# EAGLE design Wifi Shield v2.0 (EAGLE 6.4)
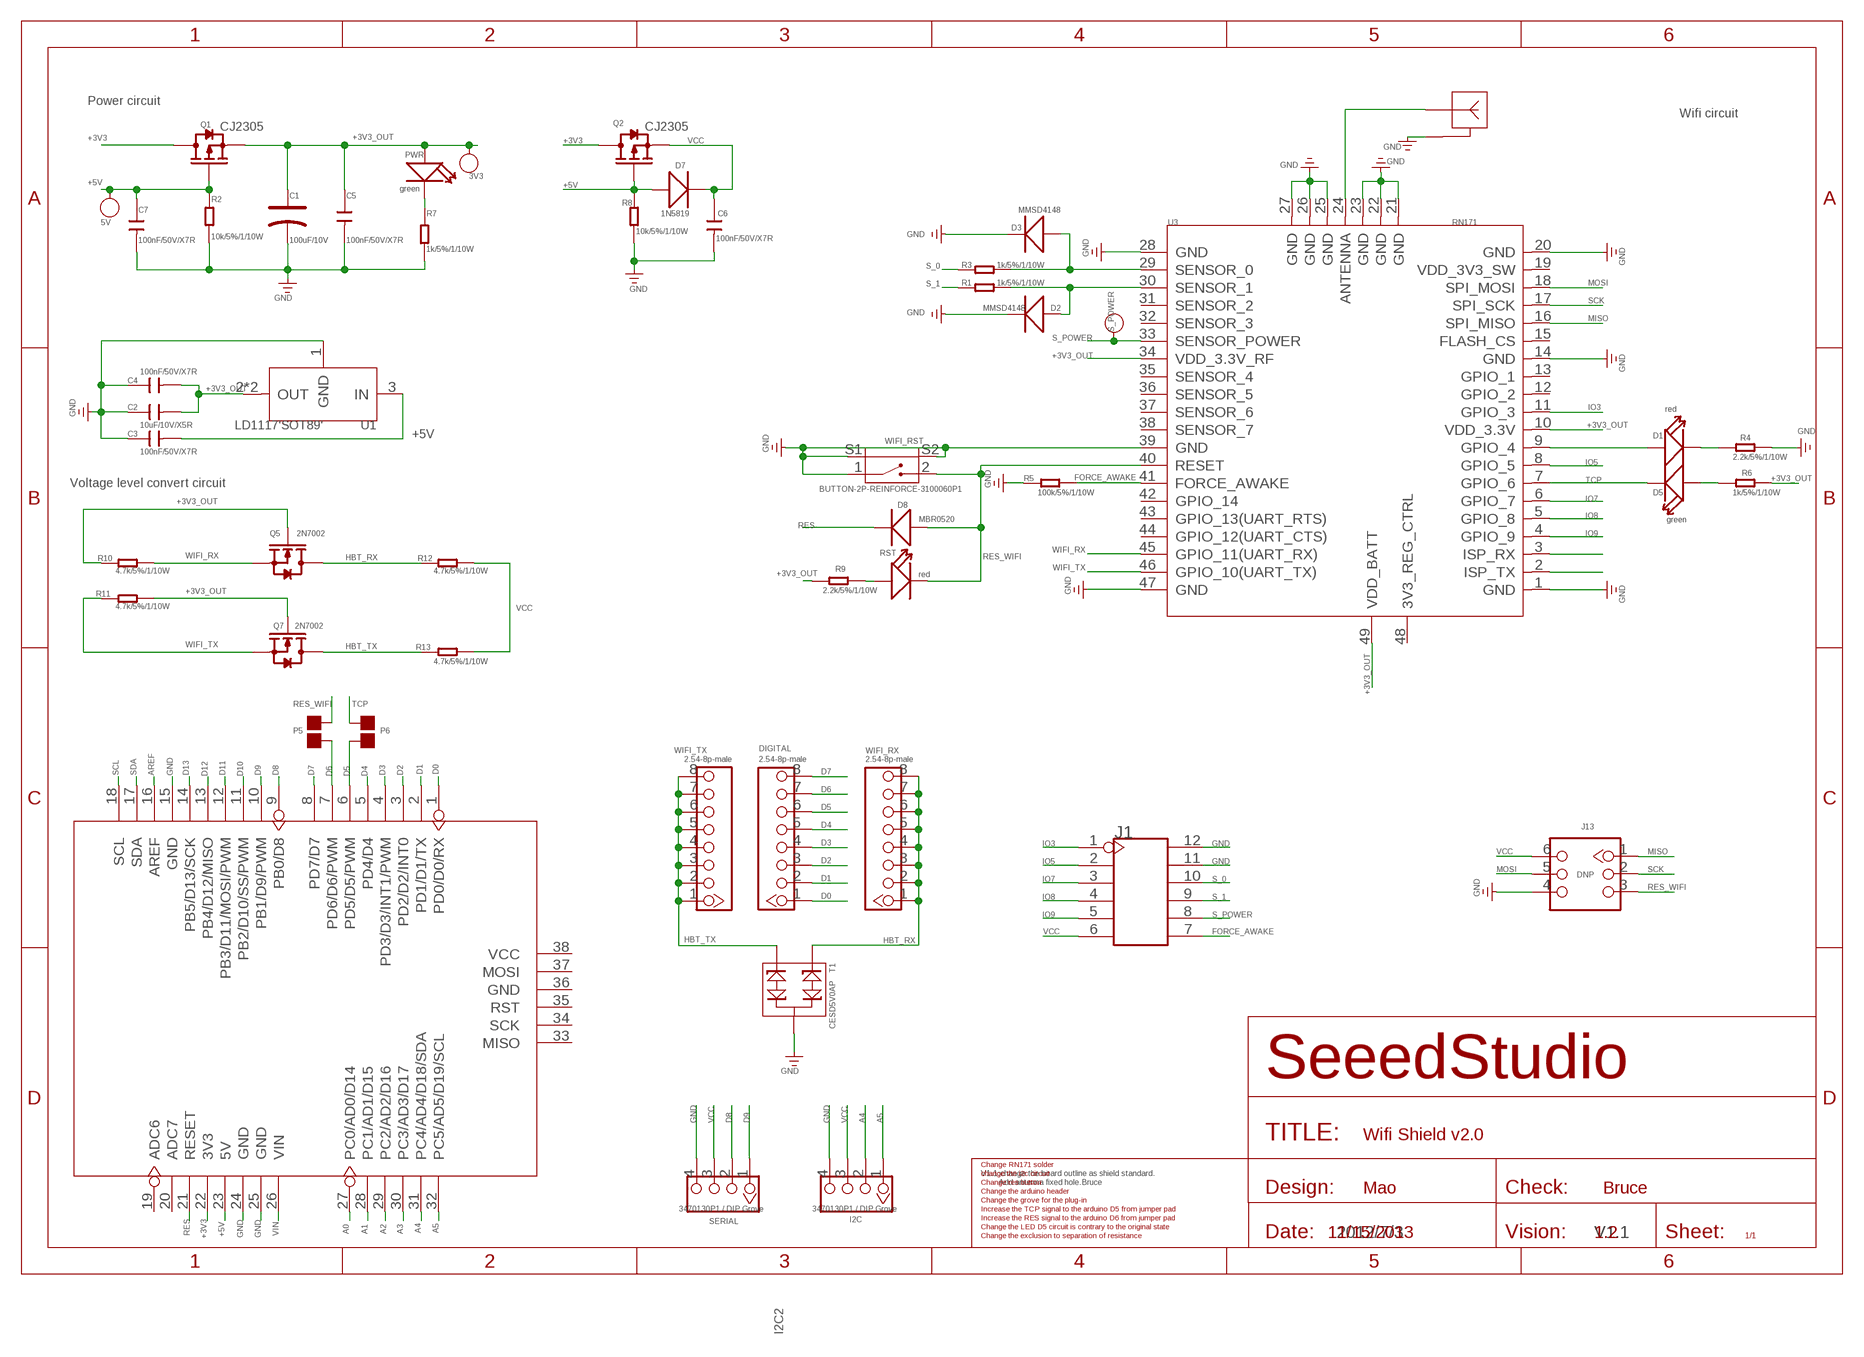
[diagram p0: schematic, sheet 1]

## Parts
3V3  PAD-TEST-POINT'4545'  [TP_4545]
5V  PAD-TEST-POINT'4545'  [TP_4545]
ANT3  2.4G-ANTNORMAL  [2.4G-ANT]
C1  100uF/10V  CAP-AVX-B  [AVX-B]
C2  10uF/10V/X5R  C-0805  [C0805]
C3  100nF/50V/X7R  C-0603  [C0603]
C4  100nF/50V/X7R  C-0603  [C0603]
C5  100nF/50V/X7R  C-0603  [C0603]
C6  100nF/50V/X7R  C-0603  [C0603]
C7  100nF/50V/X7R  C-0603  [C0603]
D1  red  LED'0603'  [LED-0603]
D2  MMSD4148  D'MBR0520LT1'  [SOD123-2.7X1.6]
D3  MMSD4148  D'MBR0520LT1'  [SOD123-2.7X1.6]
D5  green  LED'0603'  [LED-0603]
D7  1N5819  D'DO-214AC'  [D2010]
D8  MBR0520  D'MBR0520LT1'  [SOD123-2.7X1.6]
DIGITAL  2.54-8p-male  HEADER-8P-2.54  [8P-2.54]
I2C  3470130P1 / DIP Grove  TWIG-4P-2.0-2.0  [4P-2.0]
J1  HEADER-2X6P-2.54  [2X6P-2.54]
J13  DNP  HEADER-2X3P-2.54  [2X3P-2.54]
P5  DNP  PAD-JUMPER-2P  [2P-SMD-1.78X1.27]
P6  DNP  PAD-JUMPER-2P  [2P-SMD-1.78X1.27]
PWR  green  LED'0603'  [LED-0603]
Q1  CJ2305  MOSFET-P'SI2323CDS/SI2305DS<BR>'  [SOT23]
Q2  CJ2305  MOSFET-P'SI2323CDS/SI2305DS<BR>'  [SOT23]
Q5  2N7002  MOSFET-N'SOT23'  [SOT23]
Q7  2N7002  MOSFET-N'SOT23'  [SOT23]
R1  1k/5%/1/10W  R-0603  [R0603]
R2  10k/5%/1/10W  R-0603  [R0603]
R3  1k/5%/1/10W  R-0603  [R0603]
R4  2.2k/5%/1/10W  R-0603  [R0603]
R5  100k/5%/1/10W  R-0603  [R0603]
R6  1k/5%/1/10W  R-0603  [R0603]
R7  1k/5%/1/10W  R-0603  [R0603]
R8  10k/5%/1/10W  R-0603  [R0603]
R9  2.2k/5%/1/10W  R-0603  [R0603]
R10  4.7k/5%/1/10W  R-0603  [R0603]
R11  4.7k/5%/1/10W  R-0603  [R0603]
R12  4.7k/5%/1/10W  R-0603  [R0603]
R13  4.7k/5%/1/10W  R-0603  [R0603]
RST  red  LED'0603'  [LED-0603]
S_POWER  PAD-TEST-POINT'4545'  [TP_4545]
SERIAL  3470130P1 / DIP Grove  TWIG-4P-2.0-2.0  [4P-2.0]
T1  CESD5V0AP  D-ESD-PESDXL2BT  [SOT23]
U1  LD1117'SOT89'  [SOT89]
U3  RN171  WIFI-RN-171  [49P-1.27-26.67X17.78]
U6  ARDUINO-38P  [ARDUINO-38P-WITH/-SILK]
WIFI_RST  BUTTON-2P-REINFORCE-3100060P1  [4P-SMD-7.0X3.5X3.5H-90D]
WIFI_RX  2.54-8p-male  HEADER-8P-2.54  [8P-2.54]
WIFI_TX  2.54-8p-male  HEADER-8P-2.54  [8P-2.54]

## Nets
+3V3: Q1.3(D) Q2.3(D) U6.22(3V3)
+3V3_OUT: 3V3.T C1.+ C2.2 C4.2 C5.1 PWR.+ Q1.2(S) Q5.1(G) Q7.1(G) R6.1 R9.2 R10.2 R11.1 U1.2(OUT) U1.4(OUT) U3.10(VDD_3.3V) U3.34(VDD_3.3V_RF) U3.49(VDD_BATT)
+5V: 5V.T C3.2 C7.1 D7.+ Q1.1(G) Q2.1(G) R2.1 R8.1 U1.3(IN) U6.23(5V)
A0: U6.27(PC0/AD0/D14)
A1: U6.28(PC1/AD1/D15)
A2: U6.29(PC2/AD2/D16)
A3: U6.30(PC3/AD3/D17)
A4: I2C.2 U6.31(PC4/AD4/D18/SDA)
A5: I2C.1 U6.32(PC5/AD5/D19/SCL)
AREF: U6.16(AREF)
D0: DIGITAL.1 U6.1(PD0/D0/RX)
D1: DIGITAL.2 U6.2(PD1/D1/TX)
D2: DIGITAL.3 U6.3(PD2/D2/INT0)
D3: DIGITAL.4 U6.4(PD3/D3/INT1/PWM)
D4: DIGITAL.5 U6.5(PD4/D4)
D5: DIGITAL.6 P6.2 U6.6(PD5/D5/PWM)
D6: DIGITAL.7 P5.1 U6.7(PD6/D6/PWM)
D7: DIGITAL.8 U6.8(PD7/D7)
D8: SERIAL.2 U6.9(PB0/D8)
D9: SERIAL.1 U6.10(PB1/D9/PWM)
D10: U6.11(PB2/D10/SS/PWM)
D11: U6.12(PB3/D11/MOSI/PWM)
D12: U6.13(PB4/D12/MISO)
D13: U6.14(PB5/D13/SCK)
FORCE_AWAKE: J1.7 R5.1 U3.41(FORCE_AWAKE)
GND: ANT3.1 C1.- C2.1 C3.1 C4.1 C5.2 C6.2 C7.2 D2.2(-) D3.2(-) I2C.4 J1.11 J1.12 J13.4 R2.2 R4.1 R5.2 R7.1 R8.2 SERIAL.4 T1.3 U1.1(GND) U3.1(GND) U3.14(GND) U3.20(GND) U3.21(GND) U3.22(GND) U3.23(GND) U3.25(GND) U3.26(GND) U3.27(GND) U3.28(GND) U3.39(GND) U3.47(GND) U6.15(GND) U6.24(GND) U6.25(GND) WIFI_RST.1 WIFI_RST.S1 WIFI_RST.S2
HBT_RX: Q5.3(D) R12.2 T1.1 WIFI_RX.1 WIFI_RX.2 WIFI_RX.3 WIFI_RX.4 WIFI_RX.5 WIFI_RX.6 WIFI_RX.7 WIFI_RX.8
HBT_TX: Q7.3(D) R13.2 T1.2 WIFI_TX.1 WIFI_TX.2 WIFI_TX.3 WIFI_TX.4 WIFI_TX.5 WIFI_TX.6 WIFI_TX.7 WIFI_TX.8
IO3: J1.1 U3.11(GPIO_3)
IO5: J1.2 U3.8(GPIO_5)
IO7: J1.3 U3.6(GPIO_7)
IO8: J1.4 U3.5(GPIO_8)
IO9: J1.5 U3.4(GPIO_9)
MISO: J13.1 U3.16(SPI_MISO)
MOSI: J13.5 U3.18(SPI_MOSI)
N$1: R9.1 RST.+
N$2: D3.1(+) R3.1 U3.29(SENSOR_0)
N$3: D2.1(+) R1.1 U3.30(SENSOR_1)
N$4: D5.+ R6.2
N$6: ANT3.2 U3.24(ANTENNA)
N$10: U3.2(ISP_TX)
N$11: U3.3(ISP_RX)
N$22: D1.+ U3.9(GPIO_4)
N$25: D1.- R4.2
N$26: PWR.- R7.2
RES: D8.2(-) U6.21(RESET)
RES_WIFI: D8.1(+) J13.3 P5.2 RST.- U3.40(RESET) WIFI_RST.2
S_0: J1.10 R3.2
S_1: J1.9 R1.2
S_POWER: J1.8 S_POWER.T U3.33(SENSOR_POWER)
SCK: J13.2 U3.17(SPI_SCK)
SCL: U6.18(SCL)
SDA: U6.17(SDA)
TCP: D5.- P6.1 U3.7(GPIO_6)
VCC: C6.1 D7.- I2C.3 J1.6 J13.6 Q2.2(S) R12.1 R13.1 SERIAL.3
VIN: U6.26(VIN)
WIFI_RX: Q5.2(S) R10.1 U3.45(GPIO_11(UART_RX))
WIFI_TX: Q7.2(S) R11.2 U3.46(GPIO_10(UART_TX))
Unconnected: U3.12(GPIO_2) U3.13(GPIO_1) U3.15(FLASH_CS) U3.19(VDD_3V3_SW) U3.31(SENSOR_2) U3.32(SENSOR_3) U3.35(SENSOR_4) U3.36(SENSOR_5) U3.37(SENSOR_6) U3.38(SENSOR_7) U3.42(GPIO_14) U3.43(GPIO_13(UART_RTS)) U3.44(GPIO_12(UART_CTS)) U3.48(3V3_REG_CTRL) U6.19(ADC6) U6.20(ADC7) U6.33(MISO) U6.34(SCK) U6.35(RST) U6.36(GND) U6.37(MOSI) U6.38(VCC)

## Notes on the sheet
- Power circuit
- Wifi circuit
- Voltage level convert circuit
- Change RN171 solder
- change the i2c circuit | V1.1:change the board outline as shield standard.
- Change res button | Add antenna fixed hole.Bruce
- Change the arduino header | Mao | Bruce
- Change the grove for the plug-in
- Increase the TCP signal to the arduino D5 from jumper pad
- Increase the RES signal to the arduino D6 from jumper pad
- Change the LED D5 circuit is contrary to the original state
- Change the exclusion to separation of resistance | 11/15/2013 | 2012/7/3 | 1.2 | V1.1
- I2C2

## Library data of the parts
3V3 5V S_POWER = Discrete:PAD-TEST-POINT; PARTNO: DNP
ANT3 = template:2.4G-ANT
C1 = Discrete:CAP*: Electrolytic Capacitors,Tantalum Capacitors and Super Capacitors
C2-C7 = Discrete:C*: Ceramic Capacitors
D1 D5 PWR RST = Discrete:LED*
D2 D3 D7 D8 = Discrete:D*
DIGITAL WIFI_RX WIFI_TX = Connector:HEADER-8P
I2C SERIAL = Connector:TWIG-4P-2.0
J1 = Connector :HEADER-2X6P
J13 = Connector:HEADER-2X3P
P5 P6 = Discrete:PAD-JUMPER-2P; PARTNO: DNP
Q1 Q2 = Discrete:MOSFET-P
Q5 Q7 = Discrete:MOSFET-N: IRLL014: http://www.vishay.com/docs/91319/sihll014.pdf
R1-R13 = Discrete:R*
T1 = Discrete:D-ESD-PESDXL2BT
U1 = IC:LD1117: Low Drop Fixed And Adjustable Positive Voltage Regulators http://www.datasheetcatalog.org/datasheet/SGSThomsonMicroelectronics/mXuqtqv.pdf
U3 = moudle:WIFI-RN-171: WIFLY GSX 802.11 b/g wireless LAN Module
U6 = moudle:ARDUINO-38P
WIFI_RST = Discrete:BUTTON-2P-REINFORCE: TS-1188E http://www.best-dz.com/?thread-374-2.html SMD Button

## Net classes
0 default: width 0.003 mm, drill 0.254 mm, clearance 0.152 mm

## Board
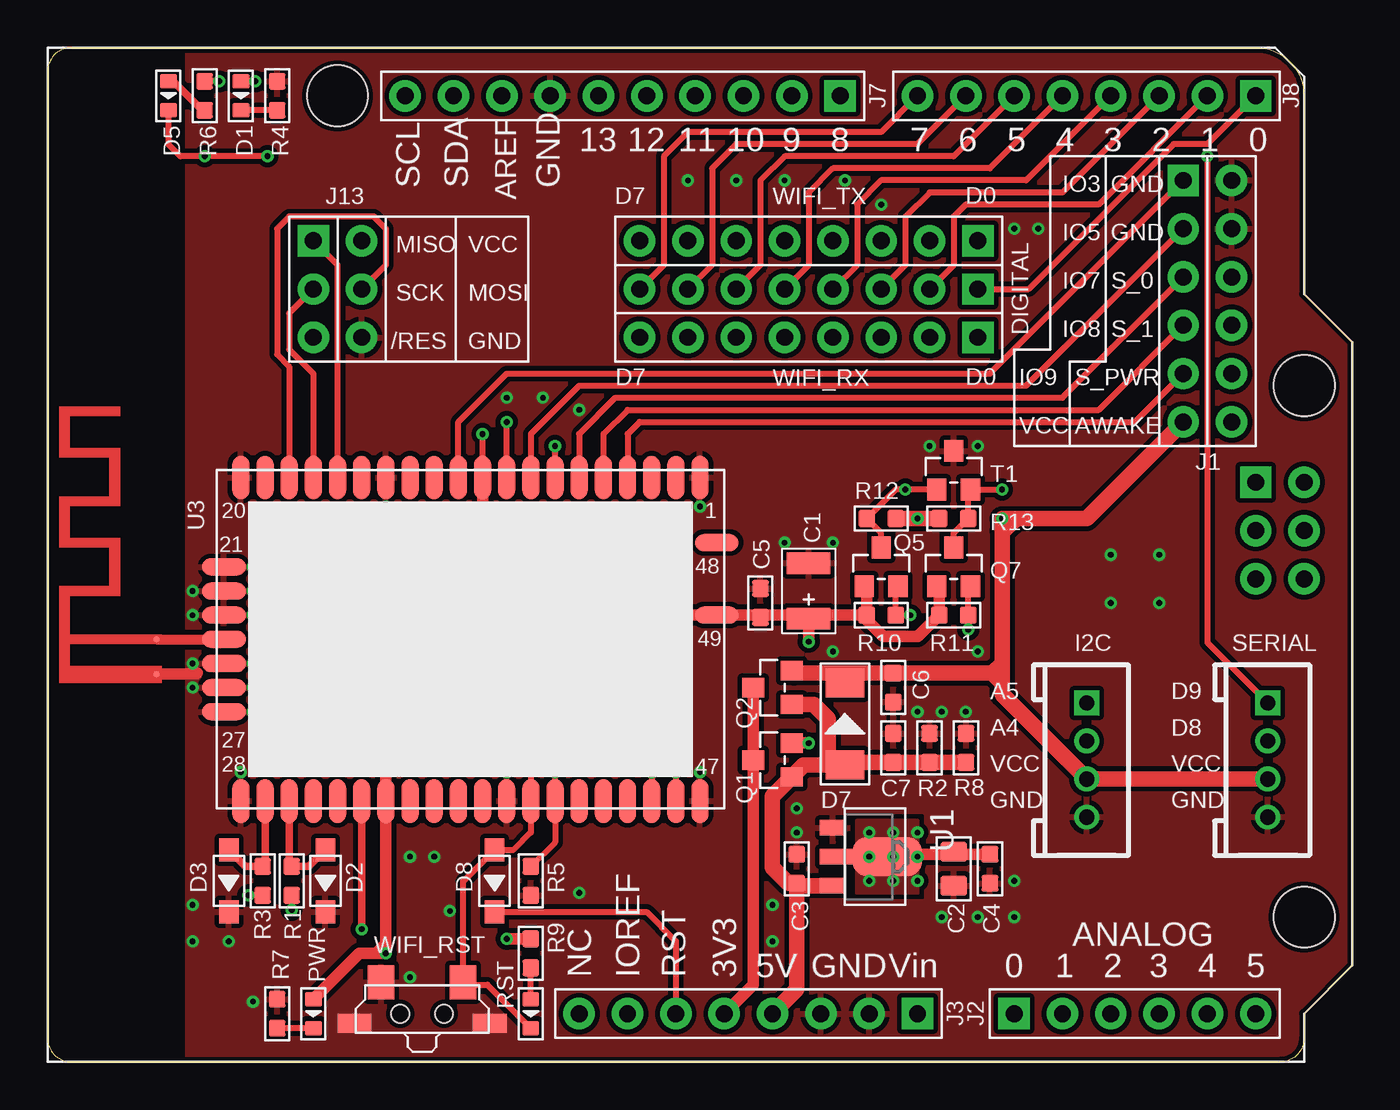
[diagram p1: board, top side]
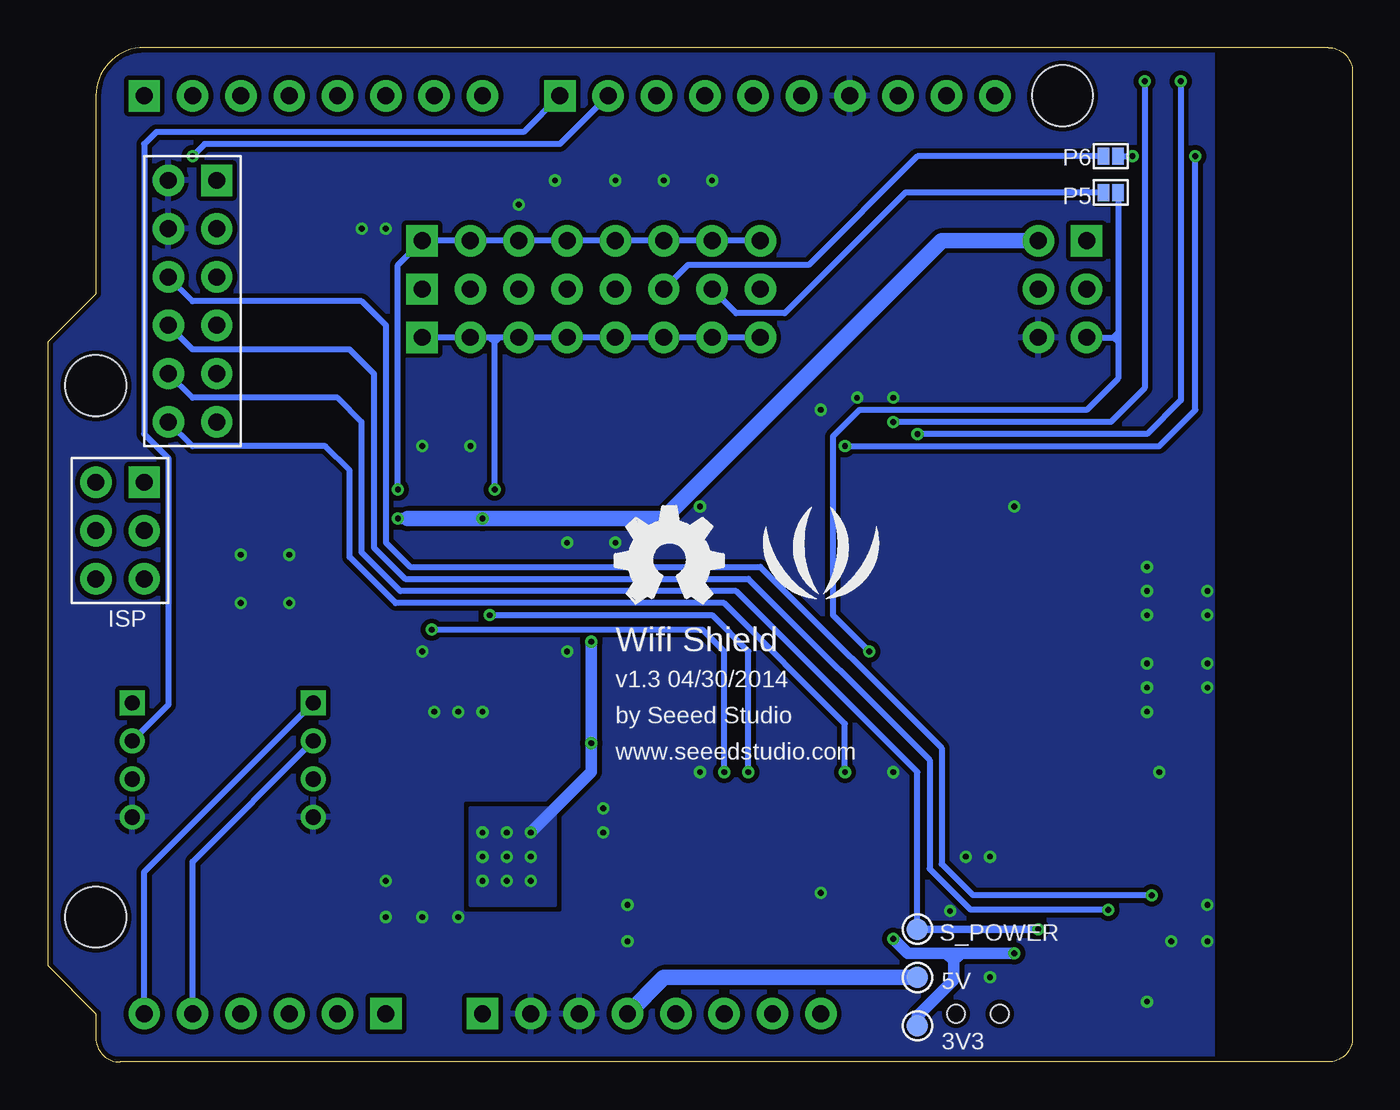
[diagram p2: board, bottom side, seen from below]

Size 68.58 x 53.34 mm. Coordinates in mm from the lower left corner, seen from the top.
Outline: 1.27,53.34 63.5,53.34 arc-90 66.04,50.8 66.04,40.39 68.58,37.85 68.58,5.08 66.04,2.54 66.04,1.27 arc-90 64.77,0 1.27,0 arc-90 0,1.27 0,52.07 arc-90 1.27,53.34
Copper layers (1*16): Top 0.035mm / dielectric 1.5mm / Bottom 0.035mm
Design rules "default": minimum track width 6mil, minimum drill 12mil, track to track 6mil, track to pad 6mil, pad to pad 6mil, via to via 6mil, smd to smd 0mil, copper to edge 10mil, drill to drill 10mil, minimum pad ring 10mil, minimum via ring 6mil, stop-mask expansion 2mil, vias tented up to drill 32mil, thermal gap 10mil
tRestrict: area 0,0 to 7,53.3; area 8.6,17.9 to 9.9,21.7
bRestrict: area 0,0 to 7,53.3

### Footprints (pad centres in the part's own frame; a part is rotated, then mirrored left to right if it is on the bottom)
TP_4545 = smd 1.143 x 1.143: T 0,0
2.4G-ANT = smd 0.305 x 0.305: 1 0.457,0.254; 2 2.286,0.254
AVX-B = smd 1.143 x 2.286: + -1.46,0; - 1.46,0
C0805 = smd 1.016 x 1.397: 1 -0.889,0; 2 0.889,0
C0603 = smd 0.889 x 0.889: 1 -0.762,0; 2 0.762,0
LED-0603 = smd 0.762 x 0.889: + -0.762,0; - 0.762,0
SOD123-2.7X1.6 = smd 1.2 x 1.02: 1 -1.635,0; 2 1.635,0
D2010 = smd 1.524 x 2.032: + -2.159,0; - 2.159,0
8P-2.54 = drill 0.889 pad 1.651 square: 1 0,8.89 | drill 0.889 pad 1.651: 2 0,6.35; 3 0,3.81; 4 0,1.27; 5 0,-1.27; 6 0,-3.81; 7 0,-6.35; 8 0,-8.89
4P-2.0 = drill 0.8 pad 1.27 square: 1 -3,0 | drill 0.8 pad 1.27: 2 -1,0; 3 1,0; 4 3,0
2X6P-2.54 = drill 0.889 pad 1.651 square: 1 -1.27,6.35 | drill 0.889 pad 1.651: 2 -1.27,3.81; 3 -1.27,1.27; 4 -1.27,-1.27; 5 -1.27,-3.81; 6 -1.27,-6.35; 7 1.27,-6.35; 8 1.27,-3.81; 9 1.27,-1.27; 10 1.27,1.27; 11 1.27,3.81; 12 1.27,6.35
2X3P-2.54 = drill 0.889 pad 1.651 square: 1 -1.27,2.54 | drill 0.889 pad 1.651: 2 -1.27,0; 3 -1.27,-2.54; 4 1.27,-2.54; 5 1.27,0; 6 1.27,2.54
2P-SMD-1.78X1.27 = smd 0.889 x 0.61: 1 0,0.381; 2 0,-0.381
SOT23 = smd 1.016 x 1.143: 1 -0.889,-1.016; 2 0.889,-1.016; 3 0,1.016
R0603 = smd 0.889 x 0.889: 1 -0.762,0; 2 0.762,0
SOT89 = smd 0.8 x 1.4: 1 -1.524,-1.905; 3 1.524,-1.905 | smd 0.8 x 1.9: 2 0,-1.651 | smd 2.032 x 3.65: 4 0,0.94
49P-1.27-26.67X17.78 = smd 0.889 x 2.286: 1 12.065,8.509; 2 10.795,8.509; 3 9.525,8.509; 4 8.255,8.509; 5 6.985,8.509; 6 5.715,8.509; 7 4.445,8.509; 8 3.175,8.509; 9 1.905,8.509; 10 0.635,8.509; 11 -0.635,8.509; 12 -1.905,8.509; 13 -3.175,8.509; 14 -4.445,8.509; 15 -5.715,8.509; 16 -6.985,8.509; 17 -8.255,8.509; 18 -9.525,8.509; 19 -10.795,8.509; 20 -12.065,8.509; 28 -12.065,-8.509; 29 -10.795,-8.509; 30 -9.525,-8.509; 31 -8.255,-8.509; 32 -6.985,-8.509; 33 -5.715,-8.509; 34 -4.445,-8.509; 35 -3.175,-8.509; 36 -1.905,-8.509; 37 -0.635,-8.509; 38 0.635,-8.509; 39 1.905,-8.509; 40 3.175,-8.509; 41 4.445,-8.509; 42 5.715,-8.509; 43 6.985,-8.509; 44 8.255,-8.509; 45 9.525,-8.509; 46 10.795,-8.509; 47 12.065,-8.509 | smd 2.286 x 0.889: 21 -12.954,3.81; 22 -12.954,2.54; 23 -12.954,1.27; 24 -12.954,0; 25 -12.954,-1.27; 26 -12.954,-2.54; 27 -12.954,-3.81; 48 12.954,5.08; 49 12.954,1.27
ARDUINO-38P-WITH/-SILK = drill 0.889 pad 1.651 square: 1 63.5,50.8; 9 41.656,50.8; 26 45.72,2.54; 27 50.8,2.54; 33 63.5,30.48 | drill 0.889 pad 1.651: 2 60.96,50.8; 3 58.42,50.8; 4 55.88,50.8; 5 53.34,50.8; 6 50.8,50.8; 7 48.26,50.8; 8 45.72,50.8; 10 39.116,50.8; 11 36.576,50.8; 12 34.036,50.8; 13 31.496,50.8; 14 28.956,50.8; 15 26.416,50.8; 16 23.876,50.8; 17 21.336,50.8; 18 18.796,50.8; 19 27.94,2.54; 20 30.48,2.54; 21 33.02,2.54; 22 35.56,2.54; 23 38.1,2.54; 24 40.64,2.54; 25 43.18,2.54; 28 53.34,2.54; 29 55.88,2.54; 30 58.42,2.54; 31 60.96,2.54; 32 63.5,2.54; 34 63.5,27.94; 35 63.5,25.4; 36 66.04,25.4; 37 66.04,27.94; 38 66.04,30.48 | hole 3.2: 15.24,50.8; 66.04,35.56; 66.04,7.62
4P-SMD-7.0X3.5X3.5H-90D = smd 1.397 x 1.778: 1 -2.159,1.651; 2 2.159,1.651 | smd 1.778 x 1.016: S1 -3.556,-0.508; S2 3.556,-0.508 | hole 0.95: -1.15,0; 1.15,0

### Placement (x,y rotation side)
3V3  22.86,1.91 180 bottom
5V  22.86,4.45 0 bottom
ANT3  5.97,19.94 90 top
C1  40.01,24.77 90 top
C2  47.62,10.16 90 top
C3  39.37,10.16 270 top
C4  49.53,10.16 90 top
C5  37.47,24.13 90 top
C6  44.45,19.68 270 top
C7  44.45,16.51 90 top
D1  10.16,50.8 270 top
D2  14.61,9.53 270 top
D3  9.53,9.53 270 top
D5  6.35,50.8 270 top
D7  41.91,17.78 90 top
D8  23.5,9.53 270 top
DIGITAL  40.01,40.64 270 top
I2C  54.61,15.88 270 top
J1  60.96,40.01 0 top
J13  15.24,40.64 0 top
P5  12.7,45.72 90 bottom
P6  12.7,47.62 270 bottom
PWR  13.97,2.54 270 top
Q1  38.1,15.88 90 top
Q2  38.1,19.68 90 top
Q5  43.81,26.04 0 top
Q7  47.62,26.04 0 top
R1  12.83,9.53 270 top
R2  46.35,16.51 90 top
R3  11.3,9.53 270 top
R4  12.06,50.8 270 top
R5  25.4,9.53 270 top
R6  8.26,50.8 270 top
R7  12.06,2.54 270 top
R8  48.27,16.51 90 top
R9  25.4,5.71 90 top
R10  43.81,23.5 180 top
R11  47.62,23.5 0 top
R12  43.81,28.57 180 top
R13  47.62,28.57 0 top
RST  25.4,2.54 270 top
S_POWER  22.86,6.99 0 bottom
SERIAL  64.14,15.88 270 top
T1  47.62,31.11 0 top
U1  43.18,10.79 270 top
U3  22.23,22.23 0 top
U6  0,0 0 top
U$1  [OSHW_FILLX200_NOTEXT]  38.73,24.13 0 bottom
U$2  [LOGO_SILK]  27.94,26.04 0 bottom
WIFI_RST  19.68,2.54 0 top
WIFI_RX  40.01,38.1 270 top
WIFI_TX  40.01,43.18 270 top

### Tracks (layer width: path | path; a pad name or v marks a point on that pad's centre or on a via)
+3V3
  Top 0.61: Q2.3 Q1.3 37.08,4.06 U6.22
+3V3_OUT  (via drill 0.3 pad 0.64)
  Top 0.203: U1.2 v43.18,10.79
  Top 0.305: U3.10 v22.86,33.02 | v9.02,51.56 R6.1
  Top 0.61: C4.2 47.75,10.92 | 47.75,10.92 C2.2 | 47.75,10.92 44.25,10.92 | 17.78,6.22 U3.34 17.78,18.41 22.86,23.5 | 17.78,6.22 v17.78,5.71 17.27,5.71 | 37.34,23.5 U3.49 23.37,23.5 | 37.34,23.5 C5.1 | 37.34,23.5 39.81,23.5 | 39.81,23.5 C1.+ v40.01,22.1 | 39.81,23.5 42.93,23.5 | 42.93,23.5 R10.2 43.05,24.89 Q5.1 | Q7.1 46.86,24.89 R11.1 45.73,22.37 43.93,22.37 42.93,23.37 42.93,23.5 | R9.2 v24.13,6.48 | PWR.+ 16.38,5.71 17.27,5.71 | Q1.2 v40.01,16.76 | 23.37,23.5 22.86,23.5 | U3.10 22.86,24 | 22.86,24 22.86,23.5 | 23.37,23.5 22.86,24 | 17.27,5.71 17.78,6.22
  Bottom 0.305: v9.02,51.56 9.02,34.8 10.79,33.02 v22.86,33.02
  Bottom 0.61: 3V3.T 22.86,2.41 20.95,4.32 20.95,5.33 | v17.78,5.71 20.95,5.71 | 20.95,5.71 21.34,5.71 | 21.34,5.71 23.37,5.71 v24.13,6.48 | 20.95,5.33 20.95,5.71 | v40.01,22.1 v40.01,16.76 40.01,15.24 v43.18,12.06 | 20.95,5.33 20.7,5.59 | 20.95,5.33 21.34,5.71
  other vias: 44.45,12.06 44.45,9.53 43.18,9.53 44.45,10.79 45.72,9.53 45.72,10.79 45.72,12.06
  pour Top (isolate 0.254, no thermals): 42.55,12.7 45.72,12.7 45.72,8.89 42.55,8.89
  pour Bottom (isolate 0.254, no thermals): 41.91,13.34 46.35,13.34 46.35,8.26 41.91,8.26
+5V
  Top 0.813: R8.1 R2.1 C7.1 42.04,15.75 D7.+ 41.02,15.62 | Q2.1 40.26,18.8 41.02,18.03 41.02,15.62 | 41.02,15.62 39.75,15.62 Q1.1 38.1,13.97 38.1,10.22 38.92,9.4 C3.2 | U6.23 39.37,3.81 C3.2 | U1.3 39.5,9.27 C3.2
  Bottom 0.813: 5V.T 36.2,4.45 U6.23
A4
  Bottom 0.305: U6.31 60.96,10.53 I2C.2
A5
  Bottom 0.305: U6.32 63.5,9.98 I2C.1
D0
  Top 0.305: U6.1 60.96,48.26 59.18,48.26 51.56,40.64 DIGITAL.1
D1
  Top 0.305: U6.2 55.24,45.09 48.26,45.09 47.62,44.45 47.62,41.91 DIGITAL.2
D2
  Top 0.305: U6.3 53.34,45.72 46.35,45.72 45.09,44.45 45.09,41.91 DIGITAL.3
D3
  Top 0.305: U6.4 51.44,46.35 43.81,46.35 42.55,45.09 42.55,41.91 DIGITAL.4
D4
  Top 0.305: U6.5 49.53,46.99 41.27,46.99 40.01,45.72 40.01,41.91 DIGITAL.5
D5
  Top 0.305: U6.6 47.62,47.62 38.73,47.62 37.47,46.35 37.47,41.91 DIGITAL.6
  Bottom 0.305: P6.2 22.86,47.62 28.57,41.91 34.92,41.91 DIGITAL.6
D6
  Top 0.305: DIGITAL.7 34.92,41.91 34.92,46.99 36.2,48.26 45.72,48.26 U6.7
  Bottom 0.305: P5.1 23.5,45.72 29.84,39.37 32.38,39.37 DIGITAL.7
D7
  Top 0.305: DIGITAL.8 32.38,41.91 32.38,47.62 33.66,48.9 43.81,48.9 U6.8
D8
  Bottom 0.305: U6.9 43.56,48.9 62.87,48.9 63.5,48.26 63.5,33.02 62.23,31.75 62.23,18.78 SERIAL.2
D9  (via drill 0.3 pad 0.64)
  Top 0.305: SERIAL.1 60.96,22.05 v60.96,47.62
  Bottom 0.305: U6.10 41.66,48.26 60.33,48.26 v60.96,47.62
FORCE_AWAKE  (via drill 0.3 pad 0.64)
  Top 0.305: v26.67,15.24 U3.41 26.67,11.56 R5.1
  Bottom 0.305: J1.7 60.96,32.38 53.98,32.38 52.7,31.11 52.7,26.54 50.29,24.13 33.02,24.13 26.67,17.78 v26.67,15.24
GND  (via drill 0.3 pad 0.64)
  Top 0.61: ANT3.1 7.82,20.4 7.87,20.45
  other vias: 46.99,18.41 48.26,18.41 41.27,27.3 38.73,27.3 7.62,6.35 9.53,6.35 10.79,3.17 19.05,4.45 27.94,8.89 39.37,12.06 39.37,13.34 50.8,9.53 48.9,7.62 50.8,7.62 46.99,7.62 45.72,18.41 24.13,34.92 26.04,34.92 10.79,26.04 41.27,21.59 48.9,21.59 17.78,29.21 19.05,10.79 33.66,46.35 36.2,46.35 38.73,46.35 41.91,46.35 43.81,45.09 50.8,43.81 52.07,43.81 27.94,34.29 55.88,24.13 58.42,24.13 58.42,26.67 55.88,26.67 46.35,32.38 48.9,32.38 38.1,8.26 38.1,6.35 20.32,10.79 21.15,7.94 24.13,15.24 34.29,15.24 34.29,29.21 10.79,24.77 10.79,23.5 10.79,20.95 10.79,19.68 10.79,18.41 10.16,15.24 7.62,8.26 7.62,20.95 7.62,19.68 7.62,23.5 7.62,24.77
  pour Top (isolate 0.254, rank 6): 0,53.34 68.58,53.34 68.58,0 0,0
  pour Bottom (isolate 0.254, rank 6): 0,53.34 68.58,53.34 68.58,0 0,0
HBT_RX  (via drill 0.3 pad 0.64)
  Top 0.305: Q5.3 43.81,27.81 R12.2 44.58,30.1 v45.09,30.1 T1.1
  Bottom 0.305: WIFI_RX.8 WIFI_RX.7 WIFI_RX.6 WIFI_RX.5 WIFI_RX.4 WIFI_RX.3 44.83,38.1 | 44.83,38.1 44.96,38.1 | 44.96,38.1 45.34,38.1 | 45.34,38.1 WIFI_RX.2 WIFI_RX.1 | v45.09,30.1 45.09,37.85 | 45.09,37.85 45.09,37.97 44.96,38.1 | 45.09,37.85 44.83,38.1 | 45.09,37.85 45.34,38.1
HBT_TX  (via drill 0.3 pad 0.64)
  Top 0.305: Q7.3 47.62,27.81 R13.2 48.39,29.97 T1.2 v50.16,30.1
  Bottom 0.305: WIFI_TX.8 WIFI_TX.7 WIFI_TX.6 WIFI_TX.5 WIFI_TX.4 WIFI_TX.3 WIFI_TX.2 WIFI_TX.1 49.78,42.29 50.16,41.91 v50.16,30.1
IO3
  Top 0.305: J1.1 49.53,36.2 24.13,36.2 21.59,33.66 U3.11
IO5
  Top 0.305: U3.8 25.4,33.02 27.94,35.56 51.44,35.56 J1.2
IO7
  Top 0.305: U3.6 27.94,33.02 29.84,34.92 53.34,34.92 J1.3
IO8
  Top 0.305: U3.5 29.21,33.02 30.48,34.29 55.24,34.29 J1.4
IO9
  Top 0.305: U3.4 30.48,33.02 31.11,33.66 57.15,33.66 J1.5
MISO
  Top 0.305: U3.16 15.24,41.91 J13.1
MOSI
  Top 0.305: J13.5 17.78,41.91 17.78,43.81 17.14,44.45 12.7,44.45 12.06,43.81 12.06,37.21 12.7,36.58 U3.18
N$1
  Top 0.305: RST.+ R9.1
N$2
  Top 0.406: U3.29 11.43,10.41 R3.1 10.4,10.29 D3.1
N$3
  Top 0.406: U3.30 12.7,10.41 R1.1 13.73,10.29 D2.1
N$4
  Top 0.406: R6.2 8.13,50.04 6.6,51.56 D5.+
N$6
  Top 0.533: ANT3.2 U3.24
N$22  (via drill 0.3 pad 0.64)
  Top 0.305: U3.9 v24.13,33.66 | v10.92,51.56 D1.+
  Bottom 0.305: v10.92,51.56 10.92,35.43 12.7,33.66 v24.13,33.66
N$25
  Top 0.305: R4.2 D1.-
N$26
  Top 0.305: PWR.- R7.2
RES
  Top 0.305: D8.2 31.48,7.89 33.02,6.35 U6.21
RES_WIFI  (via drill 0.3 pad 0.64)
  Top 0.305: RST.- 23.11,4.06 21.84,4.06 WIFI_RST.2 | 21.84,4.32 21.84,9.51 D8.1 24.5,11.16 25.4,12.06 U3.40 v25.4,21.59
  Top 0.61: WIFI_RST.2 21.84,4.32
  Bottom 0.305: v25.4,21.59 27.3,23.5 27.3,32.89 25.91,34.29 13.97,34.29 12.32,35.94 12.32,37.85 | P5.2 12.32,38.35 | 12.32,38.35 12.32,38.23 | 12.32,38.23 12.32,37.85 | J13.3 12.57,38.1 | 12.57,38.1 12.45,38.1 12.32,38.23 | 12.57,38.1 12.32,38.35 | 12.57,38.1 12.32,37.85
S_0  (via drill 0.3 pad 0.64)
  Top 0.305: R3.2 v10.54,8.76
  Bottom 0.305: v10.54,8.76 19.94,8.76 21.59,10.41 21.59,16.51 31.11,26.04 49.53,26.04 50.8,27.3 50.8,38.73 52.07,40.01 60.96,40.01 J1.10
S_1  (via drill 0.3 pad 0.64)
  Top 0.305: R1.2 v12.83,8
  Bottom 0.305: v12.83,8 20.07,8 22.23,10.16 22.23,15.88 31.75,25.4 49.78,25.4 51.44,27.05 51.44,36.2 52.7,37.47 60.96,37.47 J1.9
S_POWER  (via drill 0.3 pad 0.64)
  Top 0.406: U3.33 v16.51,6.99
  Bottom 0.305: S_POWER.T 22.86,15.24 32.38,24.77 50.04,24.77 52.07,26.8 52.07,33.66 53.34,34.92 60.96,34.92 J1.8
  Bottom 0.406: v16.51,6.99 S_POWER.T
SCK
  Top 0.305: J13.2 12.7,39.37 12.7,37.47 13.97,36.2 U3.17
TCP  (via drill 0.3 pad 0.64)
  Top 0.305: U3.7 v26.67,32.38 | v11.56,47.62 v8.26,47.62 6.99,47.62 6.35,48.26 D5.-
  Bottom 0.305: P6.1 v11.56,47.62 | v26.67,32.38 10.16,32.38 8.26,34.29 v8.26,47.62
VCC  (via drill 0.3 pad 0.64)
  Top 0.813: 41.91,20.45 C6.1 49.66,20.45 | 41.91,20.45 39.24,20.45 Q2.2 | D7.- 41.91,20.45 | SERIAL.3 I2C.3 50.16,19.32 50.16,19.94 | R12.1 v45.72,28.57 R13.1 | 50.16,27.94 v50.16,28.57 50.93,28.57 | 50.16,27.94 50.16,20.95 | 50.93,28.57 54.61,28.57 J1.6 | 49.66,20.45 50.16,20.95 | 50.16,27.94 50.29,27.94 50.93,28.57 | 50.16,20.95 50.16,19.94 | 49.66,20.45 50.16,19.94
  Bottom 0.61: v50.16,28.57 49.66,28.57
  Bottom 0.813: J13.6 21.59,43.18 36.2,28.57 v45.72,28.57 49.66,28.57
WIFI_RX  (via drill 0.3 pad 0.64)
  Top 0.305: Q5.2 44.58,24.89 R10.1 v45.34,23.5 | v31.75,15.24 U3.45
  Bottom 0.305: v45.34,23.5 33.66,23.5 31.75,21.59 v31.75,15.24
WIFI_TX  (via drill 0.3 pad 0.64)
  Top 0.305: Q7.2 48.39,24.89 R11.2 v48.39,22.73 | v33.02,15.24 U3.46
  Bottom 0.305: v48.39,22.73 34.16,22.73 33.02,21.59 v33.02,15.24

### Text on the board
tPlace: J7 | J8 | IO3 | GND | D7 | D0 | MISO | VCC | IO5 | GND | IO7 | S_0 | SCK | MOSI | IO8 | S_1 | /RES | GND | D7 | D0 | IO9 | S_PWR | VCC | AWAKE | A5 | D9 | A4 | D8 | VCC | VCC | GND | GND | J3 | J2
bPlace: ISP | Wifi Shield | v1.3 04/30/2014 | by Seeed Studio | www.seeedstudio.com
